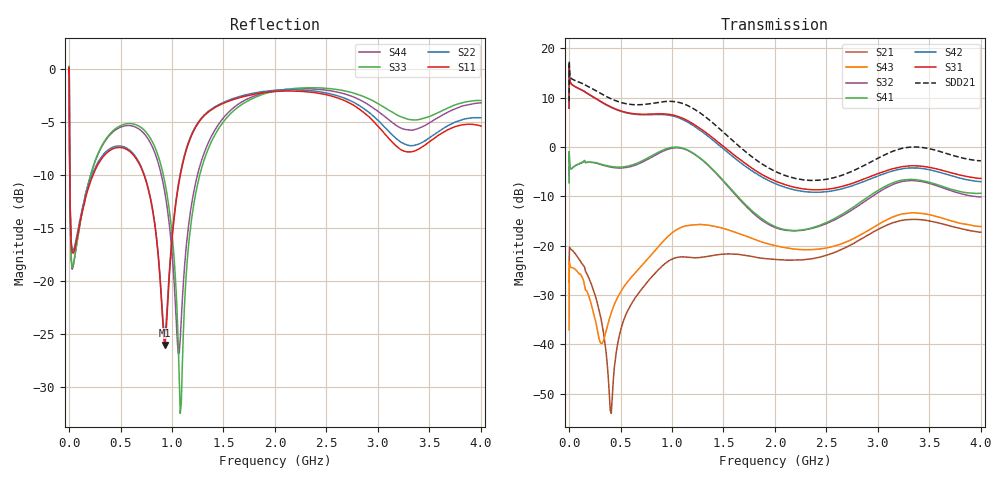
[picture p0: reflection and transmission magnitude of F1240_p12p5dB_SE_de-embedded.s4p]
! Integrated Device Technology
! Corporate Headquarters
! 6024 Silver Creek Valley Road
! San Jose, CA 95138  USA
! Phone:  1-408-284-8200
! Toll Free:  1-800-223-1366
! Webpage:  http://www.idt.com/
! Timing and RF Division
! 515 Groton Road, Suite 102
! Westford, MA 01886-6024
! Device:  F1240
! Description: Dual Intermediate Frequency Digital Variable Gain Amplifier
! Frequency:  10.0 -  500.00 MHz
! Package:  5x5 mm QFN Plastic Package: 32 pin
! Ports:  8 RF, 20 DC
!  Pin  1  = GA3 / Data  Pin 17  = RF OUT_B+
!  Pin  2  = GA4 / CLK  Pin 18  = RF OUT_B-
!  Pin  3  = GA5  Pin 19  = STBY_B
!  Pin  4  = VMODE  Pin 20  = Ground
!  Pin  5  = No Connect  Pin 21  = Ground
!  Pin  6  = GB5  Pin 22  = STB_A
!  Pin  7  = GB4  Pin 23  = RF OUT_A-  = Port 4
!  Pin  8  = GB3  Pin 24  = RF OUT_A+  = Port 3
!  Pin  9  = GB2  Pin 25  = GA0
!  Pin 10  = GB1  Pin 26  = ISET_A
!  Pin 11  = RF IN_B+  Pin 27  = VCC
!  Pin 12  = RF IN_B-  Pin 28  = Ground
!  Pin 13  = Ground  Pin 29  = RF IN_A-  = Port 2
!  Pin 14  = VCC  Pin 30  = RF IN_A+  = Port 1
!  Pin 15  = ISET_B  Pin 31  = GA1
!  Pin 16  = GB0  Pin 32  = GA2 / CSb
! Gain  = +19.5 dB
! State  = 1
! Voltage  = +5.00 V
! Current  = 85.292 mA (one channel only)
! Temperture  =  +25 C
! Test Date  =  2017-10-18
! Board  =  EB4031
! Data:  The device was measured on a custom evaluation board which has
!  individual transmission lines to the RF pins.  Data was collected
!  using a calibrated network analyzer.  The evaluation board was
!  de-embedded using Automatic Fixture Removal.
!  The reference plane is the edge of the package pin.
!  Only Channel A was measured.
!  This data is in single-ended operation.  If your needs are balanced
!  or differential S-parameters then this file needs to be used a
!  linear simulator.
! File Date:  2017-11-10  MJV
! Note:
!  Integrated Device Technology supplies this data as a sample of measured
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# Hz S dB R 100
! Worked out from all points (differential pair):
!   410 points, 500 kHz to 4 GHz, reference 100 ohm
!   strongest paths, dB at 500 kHz, 930 MHz, 1.96 GHz, 2.98 GHz, 4 GHz:
!     S31: 7.9, 6.7, -6.5, -5.6, -6.4
!     S42: 7.8, 6.5, -7.0, -6.1, -7.0
!     S41: -7.2, -0.5, -15.7, -9.1, -9.4
!     S32: -7.2, -0.7, -15.9, -9.5, -10.1
!     S43: -37.1, -18.8, -19.8, -16.0, -16.1
!     S21: -27.1, -23.7, -22.7, -16.9, -17.3
!   taken as a pair (ports 1,2 in; 3,4 out), SDD21 dB: 9.3, 9.2, -4.5, -2.5, -2.8
!   lowest |S11| = -26.0 dB at 930 MHz (marker M1), VSWR 1.11, Z = 109 + j5.26 ohm
!   |S11| at or under -10 dB: 7.296 MHz to 232.5 MHz (225.2 MHz wide, 188 % of centre); 728.4 MHz to 1.08 GHz (352 MHz wide, 38.9 % of centre)
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500000  -0.36 -5.9  -27.05 -0.4  -27.24 79.5  -59.72 68.7
        -27.05 -0.7  -0.36 -5.8  -59.51 64.6  -27.24 80.6
        7.86 -105.2  -7.20 71.0  -0.45 1.3  -37.08 -136.2
        -7.22 72.1  7.83 -104.0  -37.05 -136.0  -0.46 3.6
3000000  -3.69 -59.3  -20.78 13.0  -17.40 18.9  -41.70 65.1
         -20.77 13.1  -3.65 -59.3  -41.69 65.3  -17.41 19.0
         15.60 -176.6  -2.32 -10.0  -3.23 -55.0  -23.36 46.6
         -2.30 -9.9  15.60 -176.4  -23.31 46.4  -3.29 -54.8
2e8  -10.85 -126.0  -26.88 -89.0  -19.83 -50.8  -34.36 9.2
     -26.96 -87.5  -10.61 -127.3  -34.33 9.5  -19.86 -50.8
     10.58 109.7  -3.10 -45.3  -10.32 -88.5  -30.04 -103.8
     -3.04 -45.5  10.55 109.0  -30.75 -100.5  -10.33 -87.6
5.4e8  -7.48 -178.2  -35.65 -2.0  -21.26 -109.0  -28.29 -59.1
       -34.59 -9.2  -7.35 -179.5  -28.42 -57.4  -21.40 -109.2
       7.07 24.5  -4.21 -116.4  -5.18 -155.1  -29.81 26.9
       -4.00 -117.8  6.99 23.5  -28.09 16.8  -5.34 -154.9
9.3e8  -26.04 28.8  -23.23 -74.0  -18.94 169.2  -24.31 -151.4
       -23.65 -84.4  -24.97 26.7  -24.60 -145.9  -19.30 168.6
       6.69 -72.3  -0.70 153.6  -10.64 140.8  -19.92 -58.2
       -0.47 149.2  6.53 -74.1  -18.76 -68.9  -11.63 143.6
1.52e9  -3.12 -149.0  -21.21 147.1  -24.77 31.2  -26.28 73.3
        -21.67 150.9  -3.04 -149.0  -26.09 79.0  -25.80 30.8
        -0.24 125.5  -7.45 -29.0  -4.71 -135.4  -17.01 136.6
        -7.30 -34.1  -0.75 124.3  -16.63 132.0  -4.35 -138.4
4e9  -5.36 -154.3  -17.35 68.8  -21.09 -54.1  -20.30 -48.2
     -17.29 68.2  -4.58 -149.6  -22.22 -28.9  -23.87 -44.8
     -6.38 12.3  -10.13 -110.8  -2.95 -137.9  -15.98 88.4
     -9.38 -122.9  -7.03 21.2  -16.11 62.0  -3.16 -144.0
